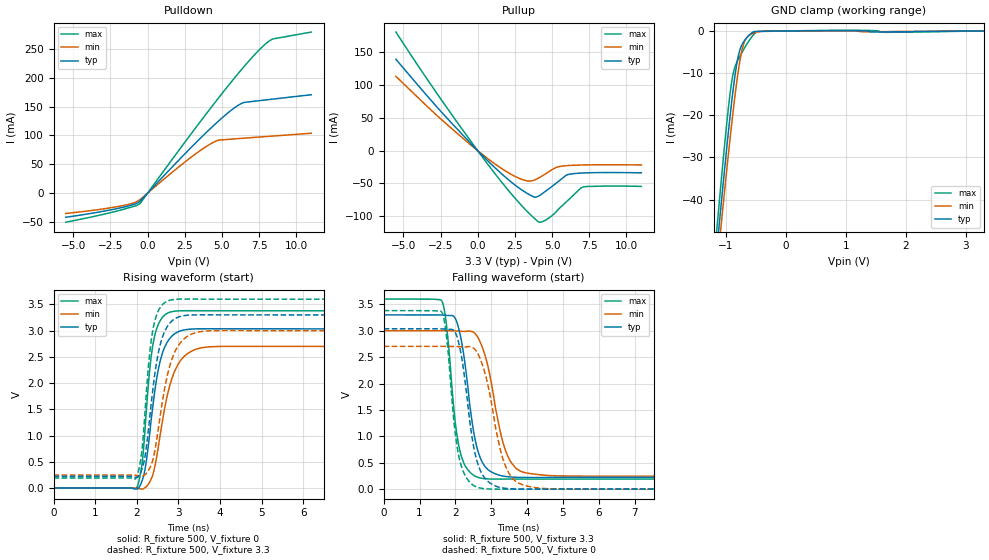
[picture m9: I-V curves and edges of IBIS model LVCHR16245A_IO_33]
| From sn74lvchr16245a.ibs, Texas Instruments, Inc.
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[Model]   LVCHR16245A_IO_33
Model_type  I/O
Vinl=0.8
Vinh=2.0
Enable   Active-Low
Vref =   0
Rref =   500
Cref =   50p
Vmeas =   1.5
| variable   typ   min   max
C_comp   5.19pF   4.50pF   6.56pF
| C_pullup   3.83pF   2.80pF   6.07pF
| C_pulldown   3.62pF   2.94pF   4.87pF
| C_tri-state   5.19pF   4.50pF   6.56pF
[Temperature Range]   40   100   -40
| Ambient temperature   25   85   -40
[Voltage range]   3.3   3   3.6
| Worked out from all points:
|   slope of the pulldown table from 0 to 0.495 V, typ, clamps not added: 36.1 ohm
|   slope of the pullup table from 0 to 0.495 V, typ, clamps not added: 43.5 ohm
|   GND clamp passes 1 mA (typ) near -0.61 V on its own axis
|   rising waveform, R_fixture 500, V_fixture 0: 20-80 % time 320ps typ, 411ps min, 227ps max; typ from 0 V to 3.03 V
|   falling waveform, R_fixture 500, V_fixture 3.3: 20-80 % time 383ps typ, 504ps min, 300ps max; typ from 3.3 V to 0.221 V
|   rising waveform, R_fixture 500, V_fixture 3.3: 20-80 % time 309ps typ, 389ps min, 224ps max; typ from 0.221 V to 3.3 V
|   falling waveform, R_fixture 500, V_fixture 0: 20-80 % time 381ps typ, 504ps min, 298ps max; typ from 3.04 V to 0 V
[GND Clamp]
| LVCHR16245A_IO_33
|   Voltage   I(typ)   I(min)   I(max)
-5.5V     -767.4mA   -751.3mA   -794.1mA
-1.15V    -52.06mA   -56.65mA   -47.21mA
-1.1V     -44.55mA   -49.38mA   -39.31mA
-1.075V   -40.85mA   -45.79mA   -35.42mA
-955mV    -23.79mA   -29.1mA    -18.09mA
-880mV    -14.27mA   -19.42mA   -10.36mA
-810mV    -7.292mA   -11.39mA   -7.246mA
-735mV    -3.396mA   -4.886mA   -5.217mA
-675mV    -2.038mA   -2.142mA   -3.74mA
-605mV    -930.6uA   -996.3uA   -2.169mA
-465mV    -89.04uA   -217.1uA   -140.9uA
3.3V      17.26pA    96.68nA    -142.7nA
[Pulldown]
| LVCHR16245A_IO_33
|   Voltage   I(typ)   I(min)   I(max)
-5.5V     -41.8mA    -35.24mA   -50.34mA
-1.885V   -25.84mA   -22.73mA   -29.86mA
-985mV    -19.86mA   -17.32mA   -23.38mA
-535mV    -14.77mA   -11.54mA   -18.38mA
2.305V    62.74mA    49.75mA    81.28mA
4.05V     107.6mA    82.56mA    141mA
4.79V     125.4mA    91.76mA    165.6mA
6.095V    152.3mA    94.47mA    207.4mA
6.5V      157.2mA    95.25mA    219.8mA
7.44V     160mA      97.05mA    246.5mA
8.3V      162.6mA    98.68mA    265.6mA
11V       170.5mA    103.7mA    279mA
[Pullup]
| LVCHR16245A_IO_33
|   Voltage   I(typ)   I(min)   I(max)
-5.5V     139.4mA    113.4mA    180.9mA
-2.18V    52.58mA    42.34mA    69.03mA
1.15V     -25.73mA   -20.03mA   -34.72mA
3.05V     -61.19mA   -44.32mA   -86.08mA
3.82V     -70.81mA   -44.67mA   -103.5mA
4.075V    -69.35mA   -41.84mA   -108.5mA
4.365V    -65.04mA   -38mA      -108mA
4.83V     -57.25mA   -31.23mA   -101.9mA
5.33V     -48.52mA   -25.09mA   -91.72mA
5.955V    -37.32mA   -22.83mA   -78.03mA
7.04V     -34.01mA   -21.75mA   -55.7mA
11V       -33.7mA    -21.66mA   -54.41mA
[Ramp]
| LVCHR16245A_IO_33
| variable   typ   min   max
dV/dt_r   1.83/3.27E-10   1.63/4.28E-10   2.04/2.32E-10
dV/dt_f   1.85/3.88E-10   1.65/5.14E-10   2.05/3.06E-10
R_load = 500
[Rising Waveform]
| LVCHR16245A_IO_33
R_fixture =   500
C_fixture =   0
L_fixture =   0
V_fixture =   0
V_fixture_min = 0
V_fixture_max = 0
|   Time   V(typ)   V(min)   V(max)
0s        346.7pV    3.772nV    7.184nV
1.995ns   -18.73mV   -5.47mV    -4.939mV
2.12ns    118.2mV    -20.08mV   417.4mV
2.19ns    314.7mV    -190.8uV   1.011V
2.31ns    1.02V      113.7mV    2.238V
2.425ns   1.797V     372.6mV    2.878V
2.635ns   2.611V     1.357V     3.268V
2.935ns   2.953V     2.267V     3.373V
3.98ns    3.036V     2.699V     3.38V
40ns      3.034V     2.699V     3.379V
[Falling Waveform]
| LVCHR16245A_IO_33
R_fixture =   500
C_fixture =   0
L_fixture =   0
V_fixture =   3.3
V_fixture_min = 3
V_fixture_max = 3.6
|   Time   V(typ)   V(min)   V(max)
0s        3.3V       3V         3.6V
1.62ns    3.298V     3V         3.566V
1.76ns    3.29V      3V         3.059V
1.98ns    3.251V     2.996V     1.37V
2.245ns   2.491V     2.987V     480.4mV
2.525ns   1.029V     2.962V     256.1mV
2.79ns    464.1mV    2.613V     199.9mV
3.485ns   232.6mV    591.5mV    189.5mV
4.44ns    220.4mV    265.8mV    190.1mV
40ns      221mV      246.2mV    190mV
[Rising Waveform]
| LVCHR16245A_IO_33
R_fixture =   500
C_fixture =   0
L_fixture =   0
V_fixture =   3.3
V_fixture_min = 3
V_fixture_max = 3.6
|   Time   V(typ)   V(min)   V(max)
0s        221mV      246.1mV    190mV
1.98ns    202.9mV    241.6mV    183.3mV
2.11ns    325.5mV    227.5mV    614.9mV
2.18ns    516mV      242.5mV    1.232V
2.3ns     1.246V     359.8mV    2.477V
2.415ns   2.056V     630.6mV    3.119V
2.615ns   2.868V     1.639V     3.494V
2.91ns    3.224V     2.584V     3.596V
3.895ns   3.301V     3.001V     3.6V
40ns      3.3V       3V         3.6V
[Falling Waveform]
| LVCHR16245A_IO_33
R_fixture =   500
C_fixture =   0
L_fixture =   0
V_fixture =   0
V_fixture_min = 0
V_fixture_max = 0
|   Time   V(typ)   V(min)   V(max)
0s        3.038V     2.704V     3.381V
1.63ns    3.035V     2.704V     3.345V
1.75ns    3.029V     2.704V     2.906V
1.965ns   3.001V     2.701V     1.248V
2.11ns    2.721V     2.697V     580.4mV
2.505ns   823.3mV    2.672V     70.43mV
2.78ns    247.5mV    2.302V     10.32mV
3.45ns    10.74mV    359.9mV    -566.3uV
4.39ns    -789.9uV   15.95mV    84.54uV
40ns      53.79uV    79.46uV    15.59uV
